ORGANIZATION_BLOCK MAIN:OB1
TITLE=Miscelatore di liquidi
//Simulatore: 10
//Versione: 1.0
//Data: 20/07/2001

BEGIN
NETWORK 1 //Imposta a 1 merker Automatico
//
LD I1.1
S M0.0 1

NETWORK 2 //Imposta a 0 merker automatico
//
LDN I1.1
R M0.0 1

NETWORK 3 //Set Marker Start in Automatico
//
LD M0.0
A I1.2
S M2.0 1

NETWORK 4 //Reset Marker Automatico
//
LDN I1.3
ON M0.0
R M2.0 1

NETWORK 5 //Imposta merker livello max
//
LD I0.4
A I0.5
= M1.2

NETWORK 6 //Imposta merker livello minimo
//
LDN I0.4
AN I0.5
= M1.0

NETWORK 7 //Contatore Quantità prodotto 1
//
LD I0.0
LD M1.0
CTU C0 +100

NETWORK 8 //Contatore Quantità prodotto 2
//
LD I0.1
LD M1.0
CTU C1 +60

NETWORK 9 //Carico prodotto 1
//
LD I1.4
AN M0.0
O M2.0
AN M1.2
AN C0
A I0.2
= Q0.0
= Q0.5

NETWORK 10 //Carico prodotto 2
//
LD I1.5
AN M0.0
O M2.0
AN M1.2
AN C1
A I0.3
= Q0.1
= Q0.6

NETWORK 11 //Memoria serbatoio Pieno
//
LD M2.0
A C1
A C0
= M2.1

NETWORK 12 //Set Marker inizio Scarico
//
LD M2.0
A I0.7
S M2.2 1

NETWORK 13 //Scarico Miscela
//
LD I1.6
AN M0.0
LD M2.0
A M2.2
OLD
AN M1.0
A I0.6
= Q0.2
= Q0.7

NETWORK 14 //Attivazione Mescolatore e Riscaldatore
//
LD I1.7
AN M0.0
LD M2.1
A I0.4
A M2.0
OLD
AN M1.0
AN I0.7
A I1.0
= Q0.4
= Q0.3

NETWORK 15 //Reset Memoria Scarico
//
LD M1.0
A M2.0
R M2.2 1

NETWORK 16 //Lampada Carico prodotto 1
//
LD Q0.0
A Q0.5
= Q1.0

NETWORK 17 //Lampada Carico prodotto 2
//
LD Q0.1
A Q0.6
= Q1.1

NETWORK 18 //Lampada segnalzione scarico
//
LD Q0.2
A Q0.7
= Q1.2

NETWORK 19 //Lampada Riscaldatore-Mescolatore
//
LD Q0.4
A Q0.3
= Q1.3

NETWORK 20 //Termico Pompa P1
//
LDN I0.2
= Q1.4

NETWORK 21 //Termico Pompa P2
//
LDN I0.3
= Q1.5

NETWORK 22 //Termico Pompa P3
//
LDN I0.6
= Q1.6

NETWORK 23 //Termico Motore Mescolatore
//
LDN I1.0
= Q1.7

END_ORGANIZATION_BLOCK

